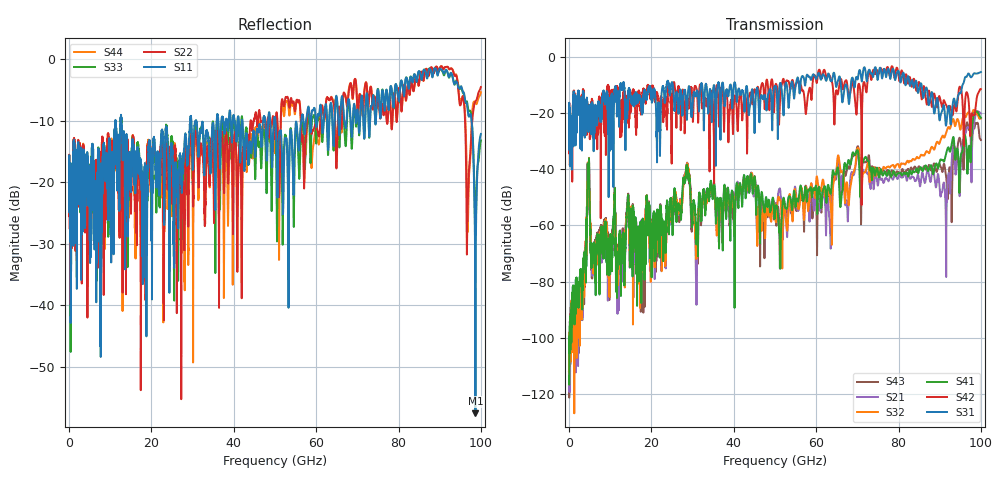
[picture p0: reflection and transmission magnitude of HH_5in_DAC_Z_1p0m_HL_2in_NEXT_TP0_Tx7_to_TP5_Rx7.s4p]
# GHz S RI R 45
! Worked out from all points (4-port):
!   4000 points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, 25 MHz to 100 GHz, reference 45 ohm
!   strongest paths, dB at 25 MHz, 25.02 GHz, 50.02 GHz, 75.03 GHz, 100 GHz:
!     S31: -18.8, -9.3, -10.5, -7.6, -5.4
!     S42: -18.8, -19.7, -11.3, -5.7, -11.5
!     S41: -113.8, -57.4, -55.6, -41.1, -21.7
!     S32: -112.1, -55.5, -54.7, -39.5, -22.0
!     S21: -116.6, -55.0, -52.5, -45.7, -20.2
!     S43: -111.8, -56.4, -53.0, -40.9, -29.6
!   lowest |S11| = -57.6 dB at 98.67 GHz (marker M1), VSWR 1.00, Z = 44.9 - j0.0566 ohm
!   |S11| at or under -10 dB: start of sweep to 11.27 GHz; 12.76 GHz to 29.39 GHz (16.64 GHz wide, 78.9 % of centre); 50.11 GHz to 56.4 GHz (6.289 GHz wide, 11.8 % of centre)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
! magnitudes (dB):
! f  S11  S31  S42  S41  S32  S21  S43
! 25 MHz  -17.1  -18.8  -18.8  -113.8  -112.1  -116.6  -111.8
! 4.725 GHz  -23.8  -26.8  -18.9  -46.2  -45.7  -46.4  -45.3
! 11.8 GHz  -14.7  -13.3  -10.9  -70.0  -76.3  -82.1  -68.5
! 28.6 GHz  -16.3  -22.4  -14.2  -39.3  -38.8  -38.7  -39.9
! 91.4 GHz  -1.8  -23.4  -16.8  -35.4  -27.8  -52.3  -40.9
! 98.67 GHz  -57.6  -6.0  -18.7  -19.8  -19.8  -20.8  -23.7
! 100 GHz  -12.2  -5.4  -11.5  -21.7  -22.0  -20.2  -29.6
